(* Logix 5000 AddOnInstructionDefinition export Banner_Q5X_3000_Param_v4; software revision 33.00; part 3 of 3 *)
(* tags used below, declared in another part *)
   Q5X : Banner_Q5X_3000_v4;
   Port_Data : Banner_IOL_Port_v4;
   Port : DINT;
   Local_Control : DINT;
   Command_Being_Processed : BOOL;
   Update_Archive : BOOL;
   Index_Write_Inprocess : INT;
   Inprocess_Index : DINT;
(* Banner_Q5X_3000_Param_v4, continued *)

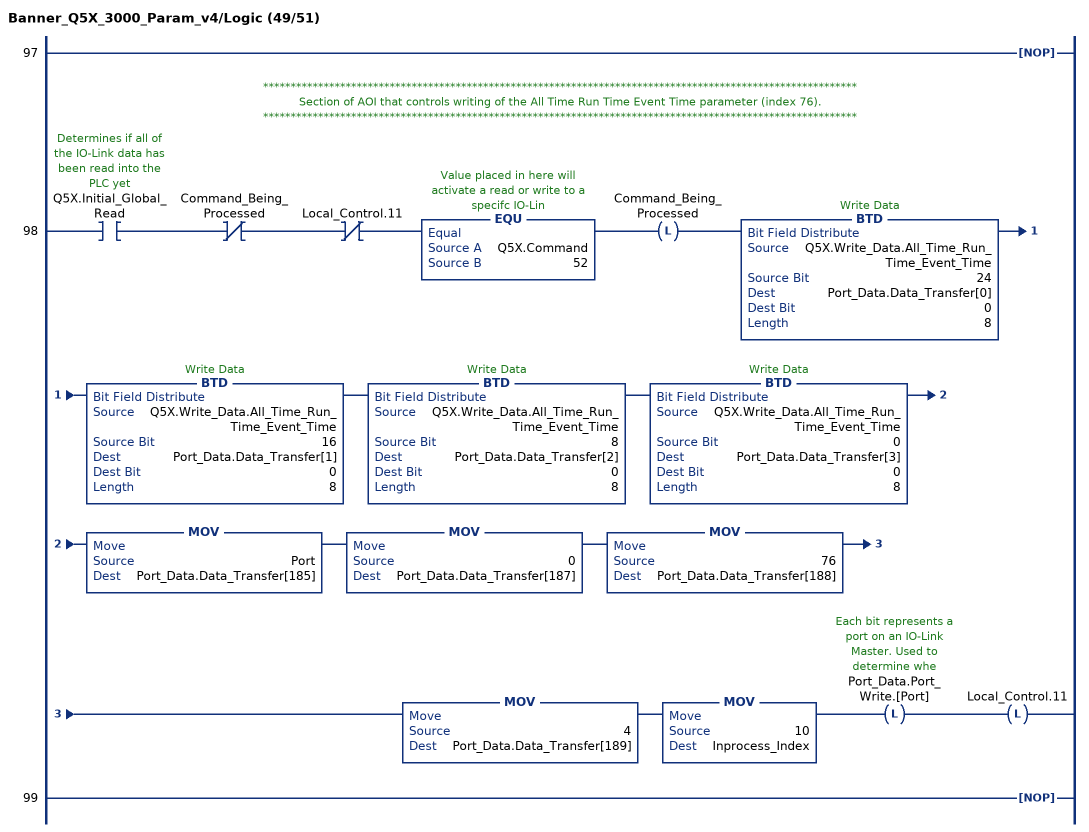
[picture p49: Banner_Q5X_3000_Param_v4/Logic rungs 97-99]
   97: NOP();
   // ************************************************************************************************************
   // Section of AOI that controls writing of the All Time Run Time Event Time parameter (index 76).
   // ************************************************************************************************************
   98: XIC(Q5X.Initial_Global_Read)XIO(Command_Being_Processed)XIO(Local_Control.11)EQU(Q5X.Command,52)OTL(Command_Being_Processed)BTD(Q5X.Write_Data.All_Time_Run_Time_Event_Time,24,Port_Data.Data_Transfer[0],0,8)BTD(Q5X.Write_Data.All_Time_Run_Time_Event_Time,16,Port_Data.Data_Transfer[1],0,8)BTD(Q5X.Write_Data.All_Time_Run_Time_Event_Time,8,Port_Data.Data_Transfer[2],0,8)BTD(Q5X.Write_Data.All_Time_Run_Time_Event_Time,0,Port_Data.Data_Transfer[3],0,8)MOV(Port,Port_Data.Data_Transfer[185])MOV(0,Port_Data.Data_Transfer[187])MOV(76,Port_Data.Data_Transfer[188])MOV(4,Port_Data.Data_Transfer[189])MOV(10,Inprocess_Index)OTL(Port_Data.Port_Write.[Port])OTL(Local_Control.11);
   99: NOP();
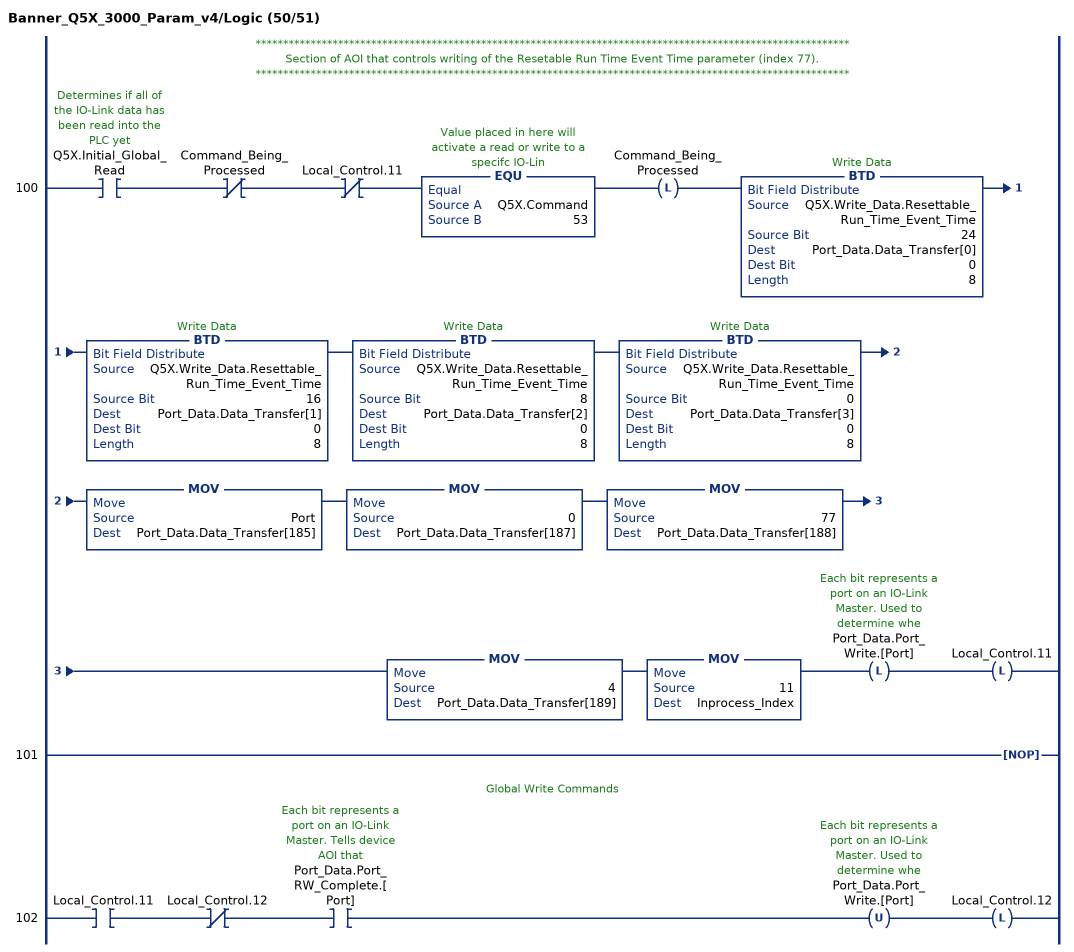
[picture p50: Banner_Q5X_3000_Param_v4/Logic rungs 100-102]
   // ************************************************************************************************************
   // Section of AOI that controls writing of the Resetable Run Time Event Time parameter (index 77).
   // ************************************************************************************************************
   100: XIC(Q5X.Initial_Global_Read)XIO(Command_Being_Processed)XIO(Local_Control.11)EQU(Q5X.Command,53)OTL(Command_Being_Processed)BTD(Q5X.Write_Data.Resettable_Run_Time_Event_Time,24,Port_Data.Data_Transfer[0],0,8)BTD(Q5X.Write_Data.Resettable_Run_Time_Event_Time,16,Port_Data.Data_Transfer[1],0,8)BTD(Q5X.Write_Data.Resettable_Run_Time_Event_Time,8,Port_Data.Data_Transfer[2],0,8)BTD(Q5X.Write_Data.Resettable_Run_Time_Event_Time,0,Port_Data.Data_Transfer[3],0,8)MOV(Port,Port_Data.Data_Transfer[185])MOV(0,Port_Data.Data_Transfer[187])MOV(77,Port_Data.Data_Transfer[188])MOV(4,Port_Data.Data_Transfer[189])MOV(11,Inprocess_Index)OTL(Port_Data.Port_Write.[Port])OTL(Local_Control.11);
   101: NOP();
   // Global Write Commands
   102: XIC(Local_Control.11)XIO(Local_Control.12)XIC(Port_Data.Port_RW_Complete.[Port])OTU(Port_Data.Port_Write.[Port])OTL(Local_Control.12);
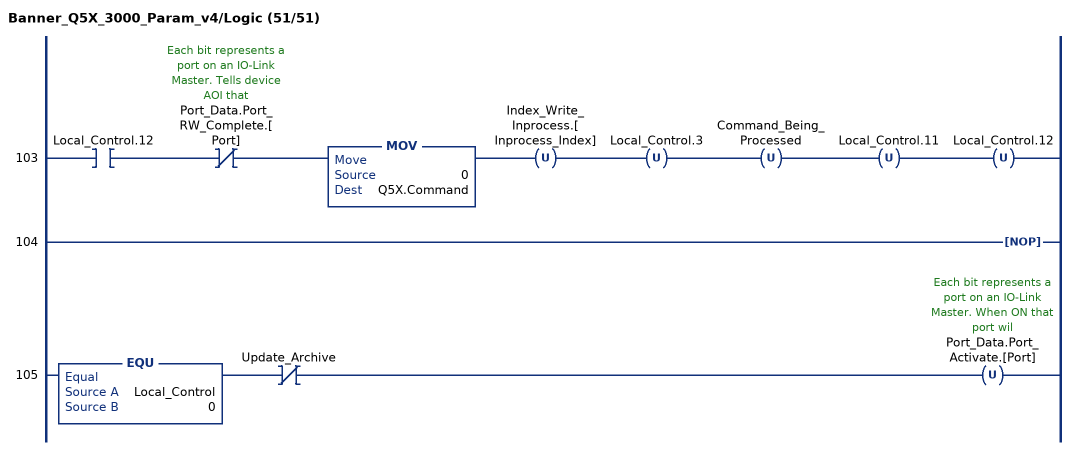
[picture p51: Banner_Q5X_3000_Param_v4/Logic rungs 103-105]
   103: XIC(Local_Control.12)XIO(Port_Data.Port_RW_Complete.[Port])MOV(0,Q5X.Command)OTU(Index_Write_Inprocess.[Inprocess_Index])OTU(Local_Control.3)OTU(Command_Being_Processed)OTU(Local_Control.11)OTU(Local_Control.12);
   104: NOP();
   105: EQU(Local_Control,0)XIO(Update_Archive)OTU(Port_Data.Port_Activate.[Port]);
END_ROUTINE
END_ADD_ON_INSTRUCTION
